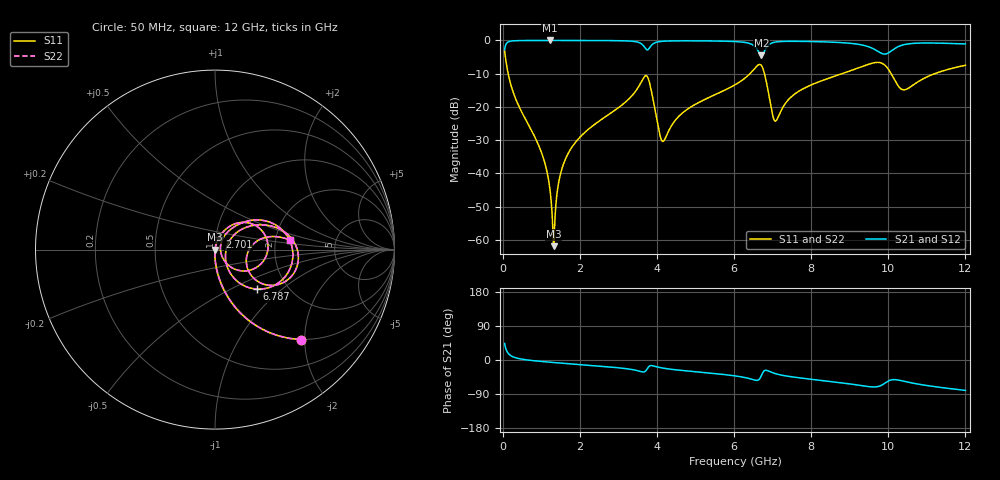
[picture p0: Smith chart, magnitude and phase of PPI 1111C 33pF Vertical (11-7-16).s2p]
# GHz S MA R 50
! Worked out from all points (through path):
!   1601 points, 50 MHz to 12 GHz, reference 50 ohm
!   highest |S21| = -0.01 dB at 1.215 GHz (marker M1); lowest = -4.5 dB at 6.712 GHz (marker M2)
!   group delay of S21, straight-line fit = 18.6 ps
!   lowest |S11| = -61.9 dB at 1.32 GHz (marker M3), VSWR 1.00, Z = 50.1 - j0.0207 ohm
!   |S11| at or under -10 dB: 142.3 MHz to 6.413 GHz (6.27 GHz wide, 191 % of centre); 6.789 GHz to 8.8 GHz (2.01 GHz wide, 25.8 % of centre); 10.07 GHz to 11.2 GHz (1.129 GHz wide, 10.6 % of centre)
!   |S22| runs from -61.9 to -3.2 dB; largest |S21 - S12| = 0
!   S11 on the Smith chart (normalised r, x): 50 MHz: 0.99, -1.91; 2.701 GHz: 1.04, +0.15; 6.787 GHz: 1.41, -0.69; 12 GHz: 2.42, +0.30
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0.05  0.6918 -46.5  0.7219 43.5  0.7219 43.5  0.6918 -46.5
0.2441875  0.1866 -80.4  0.982 9.5  0.982 9.5  0.1866 -80.4
0.9835938  0.02232 -91.9  0.999 -3.7  0.999 -3.7  0.02232 -91.9
1.215125  0.006402 -88.9  0.9991 -5.7  0.9991 -5.7  0.006402 -88.9
1.319687  0.0008046 -14.9  0.9991 -6.6  0.9991 -6.6  0.0008046 -14.9
1.558688  0.0129 77.5  0.9989 -8.6  0.9989 -8.6  0.0129 77.5
2.044156  0.03706 75.9  0.9981 -12.4  0.9981 -12.4  0.03706 75.9
2.701406  0.07359 70.5  0.9949 -17.7  0.9949 -17.7  0.07359 70.5
3.717156  0.296 5.5  0.7394 -27.9  0.7394 -27.9  0.296 5.5
4.038312  0.04867 -40.8  0.9544 -19.0  0.9544 -19.0  0.04867 -40.8
4.17275  0.0307 11.3  0.9739 -21.7  0.9739 -21.7  0.0307 11.3
4.7105  0.08541 55.6  0.9869 -28.2  0.9869 -28.2  0.08541 55.6
6.025  0.2151 44.3  0.9623 -41.9  0.9623 -41.9  0.2151 44.3
6.495531  0.3562 23.9  0.8504 -51.9  0.8504 -51.9  0.3562 23.9
6.712125  0.4177 -21.6  0.5952 -40.4  0.5952 -40.4  0.4177 -21.6
6.786812  0.3205 -43.3  0.6867 -28.2  0.6867 -28.2  0.3205 -43.3
7.070625  0.0611 -9.0  0.9447 -35.9  0.9447 -35.9  0.0611 -9.0
8.019156  0.2163 35.3  0.9622 -51.0  0.9622 -51.0  0.2163 35.3
9.654813  0.4643 -3.2  0.7274 -71.1  0.7274 -71.1  0.4643 -3.2
10.01331  0.3613 -33.4  0.6542 -54.7  0.6542 -54.7  0.3613 -33.4
10.41662  0.1809 -10.0  0.8659 -56.3  0.8659 -56.3  0.1809 -10.0
12  0.4232 7.0  0.885 -80.2  0.885 -80.2  0.4232 7.0
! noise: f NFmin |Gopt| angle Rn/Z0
0.05  0.0003337  0.8526  0.9561  0.0004826
1.372  0.003298  0.6372  6.882  0.001707
2.701  0.007599  0.6839  13.21  0.004601
4.031  0.04246  0.9058  20.03  0.09589
5.36  0.01909  0.7491  26.05  0.01456
6.682  0.1842  0.9644  32.52  1.079
8.012  0.03134  0.7791  38.13  0.026
9.341  0.07694  0.8918  44.13  0.1331
10.67  0.08271  0.8889  49.76  0.1333
12  0.0466  0.7969  54.46  0.03766
